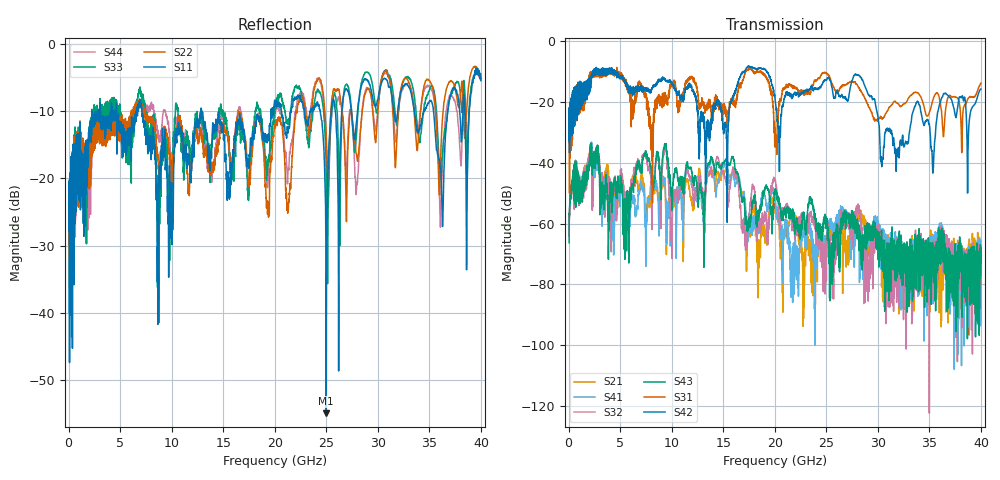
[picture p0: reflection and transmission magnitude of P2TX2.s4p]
!Agilent Technologies,N5245A,MY49151084,A.09.20.08
!Agilent N5245A: A.09.20.08
!Date: Thursday, March 01, 2012 14:34:18
!Correction: S11(Full 4 Port(1,2,3,4))
!S12(Full 4 Port(1,2,3,4))
!S13(Full 4 Port(1,2,3,4))
!S14(Full 4 Port(1,2,3,4))
!S21(Full 4 Port(1,2,3,4))
!S22(Full 4 Port(1,2,3,4))
!S23(Full 4 Port(1,2,3,4))
!S24(Full 4 Port(1,2,3,4))
!S31(Full 4 Port(1,2,3,4))
!S32(Full 4 Port(1,2,3,4))
!S33(Full 4 Port(1,2,3,4))
!S34(Full 4 Port(1,2,3,4))
!S41(Full 4 Port(1,2,3,4))
!S42(Full 4 Port(1,2,3,4))
!S43(Full 4 Port(1,2,3,4))
!S44(Full 4 Port(1,2,3,4))
!S4P File: Measurements: <S11,S12,S13,S14>,
!<S21,S22,S23,S24>,
!<S31,S32,S33,S34>,
!<S41,S42,S43,S44>:
# Hz S  dB  R 50
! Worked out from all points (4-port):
!   3996 points, 50 MHz to 40 GHz, reference 50 ohm
!   strongest paths, dB at 50 MHz, 10.04 GHz, 20.03 GHz, 30.02 GHz, 40 GHz:
!     S42: -24.6, -13.9, -19.1, -25.1, -15.7
!     S31: -24.7, -13.8, -28.4, -25.5, -13.8
!     S43: -66.3, -55.6, -48.6, -69.0, -72.8
!     S32: -64.3, -58.9, -45.7, -65.4, -71.4
!     S41: -63.0, -50.8, -51.8, -60.8, -65.5
!     S21: -63.5, -51.9, -55.7, -62.8, -76.0
!   lowest |S11| = -54.9 dB at 25 GHz (marker M1), VSWR 1.00, Z = 50 + j0.175 ohm
!   |S11| at or under -10 dB: start of sweep to 2.799 GHz; 7.106 GHz to 12.82 GHz (5.713 GHz wide, 57.3 % of centre); 12.9 GHz to 19.64 GHz (6.747 GHz wide, 41.5 % of centre)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
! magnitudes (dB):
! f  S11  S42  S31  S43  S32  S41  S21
! 50 MHz  -22.0  -24.6  -24.7  -66.3  -64.3  -63.0  -63.5
! 2.07 GHz  -12.3  -12.0  -12.2  -36.5  -37.1  -35.7  -35.8
! 5.44 GHz  -14.6  -13.4  -13.6  -60.6  -59.0  -52.8  -50.9
! 9.34 GHz  -12.7  -12.6  -19.2  -33.7  -35.0  -45.4  -46.7
! 25 GHz  -54.9  -12.8  -10.4  -58.3  -65.1  -68.1  -65.4
! 30.41 GHz  -5.6  -39.5  -25.7  -66.1  -66.2  -66.0  -69.2
! 40 GHz  -5.5  -15.7  -13.8  -72.8  -71.4  -65.5  -76.0
